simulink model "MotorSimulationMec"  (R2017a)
settings: Solver=VariableStepAuto  StartTime=0.0  StopTime=2  RelTol=1e-3
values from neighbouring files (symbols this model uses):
  a = b+al    (= 0)    [MotorSimulation.m]
  J = Jm+Jl    (= 0.000101)    [MotorSimulation.m]
  Jm = 0.0001    [MotorSimulation.m]
  Ke = 0.0019    [MotorSimulation.m]
  Kt = 0.9    [MotorSimulation.m]
  L = 0    [MotorSimulation.m]
  R = 3.75    [MotorSimulation.m]
  Td = 0.007    [MotorSimulation.m]
  Vbat = 6    [MotorSimulation.m]

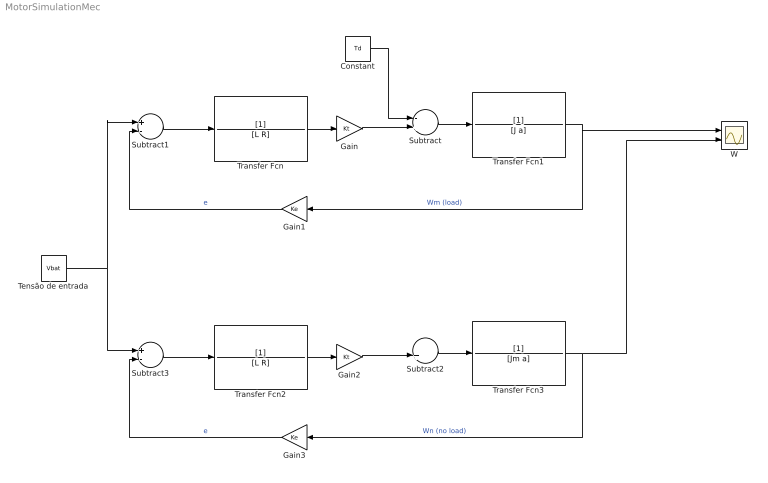
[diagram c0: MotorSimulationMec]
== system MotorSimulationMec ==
  Constant : Constant  Value=Td
  Gain : Gain  Gain=Kt
  Gain1 : Gain  Gain=Ke
  Gain2 : Gain  Gain=Kt
  Gain3 : Gain  Gain=Ke
  Subtract : Sum  Inputs=-+
  Subtract1 : Sum  Inputs=+-
  Subtract2 : Sum  Inputs=-+
  Subtract3 : Sum  Inputs=+-
  Tensão de entrada : Constant  Value=Vbat
  Transfer Fcn : TransferFcn  Denominator=[L R]
  Transfer Fcn1 : TransferFcn  Denominator=[J a]
  Transfer Fcn2 : TransferFcn  Denominator=[L R]
  Transfer Fcn3 : TransferFcn  Denominator=[Jm a]
  W : Scope  NumInputPorts=2
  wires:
  Transfer Fcn/1 -> Gain/1
  Gain/1 -> Subtract/2
  Subtract1/1 -> Transfer Fcn/1
  Tensão de entrada/1 -> Subtract1/1, Subtract3/1
  Constant/1 -> Subtract/1
  Gain1/1 -> Subtract1/2  "e"
  Subtract/1 -> Transfer Fcn1/1
  Transfer Fcn1/1 -> Gain1/1, W/1  "Wm (load)"
  Gain3/1 -> Subtract3/2  "e"
  Transfer Fcn2/1 -> Gain2/1
  Transfer Fcn3/1 -> Gain3/1, W/2  "Wn (no load)"
  Gain2/1 -> Subtract2/2
  Subtract2/1 -> Transfer Fcn3/1
  Subtract3/1 -> Transfer Fcn2/1
